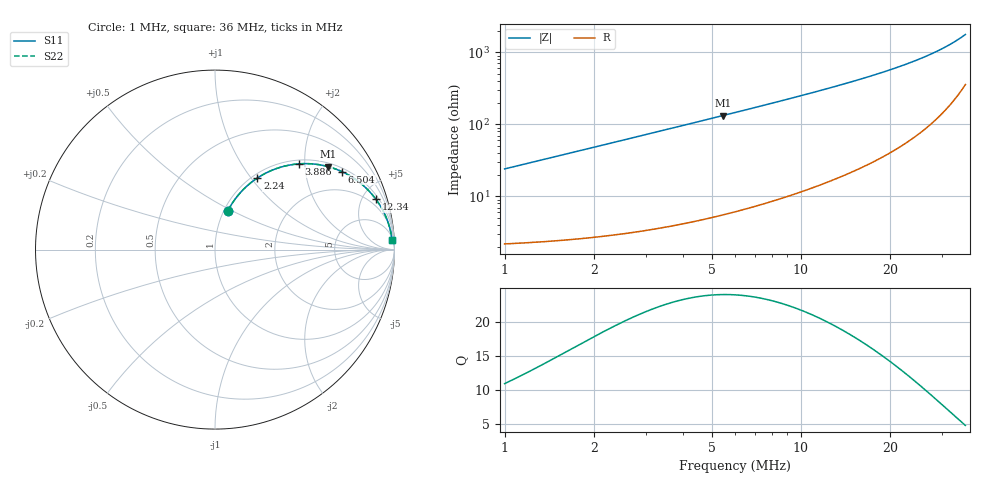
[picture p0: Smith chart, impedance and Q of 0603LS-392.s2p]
# MHz S MA R 50
!Freq  MagS11  AngS11  MagS21  AngS21  MagS12  AngS12  MagS22  AngS22
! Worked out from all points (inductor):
!   801 points, 1 MHz to 36 MHz, reference 50 ohm
!   read as one part in series: L = 3.81 uH near 1.018 MHz
!   highest Q = 23.9 at 5.461 MHz (marker M1), where L = 3.85 uH
!   S11 on the Smith chart (normalised r, x): 1 MHz: 1.04, +0.48; 2.24 MHz: 1.06, +1.07; 3.886 MHz: 1.08, +1.87; 6.504 MHz: 1.13, +3.17; 12.34 MHz: 1.32, +6.28; 36 MHz: 8, +35
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1  0.2291 71.6  0.9528 -13.2  0.9528 -13.2  0.2291 71.6
1.267959  0.2854 69.1  0.937 -16.5  0.937 -16.5  0.2854 69.1
1.551126  0.3417 66.3  0.9176 -19.9  0.9176 -19.9  0.3417 66.3
1.872203  0.4013 63.0  0.8928 -23.6  0.8928 -23.6  0.4013 63.0
2.239588  0.4635 59.4  0.8619 -27.6  0.8619 -27.6  0.4635 59.4
2.60802  0.5196 55.9  0.8292 -31.3  0.8292 -31.3  0.5196 55.9
3.009976  0.5737 52.4  0.7928 -35.0  0.7928 -35.0  0.5737 52.4
3.885524  0.6691 45.6  0.7147 -42.0  0.7147 -42.0  0.6691 45.6
4.668852  0.7331 40.5  0.65 -47.1  0.65 -47.1  0.7331 40.5
5.461329  0.7823 36.2  0.5911 -51.4  0.5911 -51.4  0.7823 36.2
6.503813  0.83 31.6  0.524 -56.0  0.524 -56.0  0.83 31.6
6.862978  0.843 30.2  0.5034 -57.4  0.5034 -57.4  0.843 30.2
7.95628  0.875 26.6  0.4477 -60.9  0.4477 -60.9  0.875 26.6
9.223751  0.9014 23.2  0.3943 -64.2  0.3943 -64.2  0.9014 23.2
10.64534  0.9223 20.2  0.3455 -67.1  0.3455 -67.1  0.9223 20.2
12.34119  0.9395 17.4  0.2986 -69.8  0.2986 -69.8  0.9395 17.4
12.67738  0.9422 16.9  0.2905 -70.2  0.2905 -70.2  0.9422 16.9
15.30154  0.9582 13.7  0.2371 -73.1  0.2371 -73.1  0.9582 13.7
18.55182  0.9699 10.8  0.1883 -75.4  0.1883 -75.4  0.9699 10.8
24.38117  0.9805 7.3  0.1281 -77.6  0.1281 -77.6  0.9805 7.3
30.22962  0.9853 4.9  0.08659 -77.7  0.08659 -77.7  0.9853 4.9
36  0.9873 3.1  0.05579 -75.2  0.05579 -75.2  0.9873 3.1
